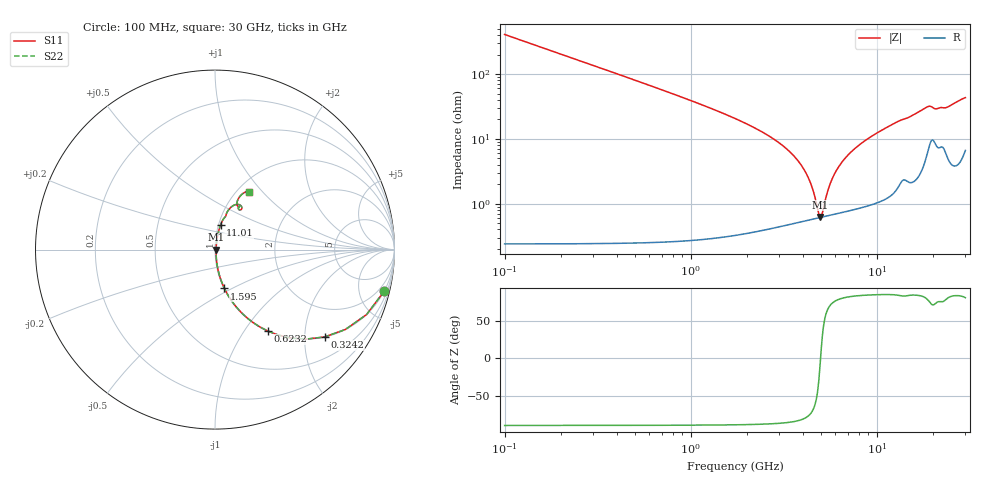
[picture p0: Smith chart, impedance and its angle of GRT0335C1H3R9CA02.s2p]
!Murata Part Number: GRT0335C1H3R9CA02
!These Parameters are Measured in Series Mode Connection
!Data Generated on Jun 19, 2026
!  o--ll--o
!Port1  Port2
!  o------o
!Operation Temp=25[degC], DC Bias Voltage=0[V]
!Freq. Start=100[MHz] Stop=30[GHz] 401[Steps]
# Hz S RI R 50
!Freq.(Hz) S11(Real) S11(Imag) S21(Real) S21(Imag) S12(Real) S12(Imag) S22(Real) S22(Imag)
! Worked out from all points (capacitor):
!   401 points, 100 MHz to 30 GHz, reference 50 ohm
!   read as one part in series: C = 3.9 pF near 249.5 MHz
!   lowest |Z| = 621 mohm at 4.959 GHz (marker M1)
!   series resonance near 4.994 GHz, so ESL is about 260 pH
!   S11 on the Smith chart (normalised r, x): 100 MHz: 1.00, -8.16; 324.2 MHz: 1.00, -2.51; 623.2 MHz: 1.01, -1.29; 1.595 GHz: 1.01, -0.46; 11.01 GHz: 1.02, +0.29; 30 GHz: 1.13, +0.85
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1e8  0.9432 -0.2312  0.0568 0.2312  0.0568 0.2312  0.9432 -0.2312
3.2425e8  0.6107 -0.4866  0.3893 0.4866  0.3893 0.4866  0.6107 -0.4866
6.2325e8  0.294 -0.4536  0.706 0.4536  0.706 0.4536  0.294 -0.4536
9.97e8  0.1351 -0.3385  0.8649 0.3385  0.8649 0.3385  0.1351 -0.3385
1.595e9  0.0525 -0.2162  0.9475 0.2162  0.9475 0.2162  0.0525 -0.2162
3.16475e9  0.0103 -0.0753  0.9897 0.0753  0.9897 0.0753  0.0103 -0.0753
3.91225e9  0.00676 -0.0393  0.9932 0.0393  0.9932 0.0393  0.00676 -0.0393
4.36075e9  0.00606 -0.0217  0.9939 0.0217  0.9939 0.0217  0.00606 -0.0217
4.80925e9  0.00599 -0.00601  0.994 0.00601  0.994 0.00601  0.00599 -0.00601
4.95875e9  0.00607 -0.00114  0.9939 0.00114  0.9939 0.00114  0.00607 -0.00114
5.10825e9  0.0062 0.00359  0.9938 -0.00359  0.9938 -0.00359  0.0062 0.00359
5.482e9  0.0067 0.0148  0.9933 -0.0148  0.9933 -0.0148  0.0067 0.0148
5.70625e9  0.0071 0.0212  0.9929 -0.0212  0.9929 -0.0212  0.0071 0.0212
6.60325e9  0.00934 0.0448  0.9907 -0.0448  0.9907 -0.0448  0.00934 0.0448
8.0235e9  0.0145 0.0775  0.9855 -0.0775  0.9855 -0.0775  0.0145 0.0775
1.01165e10  0.025 0.12  0.975 -0.12  0.975 -0.12  0.025 0.12
1.10135e10  0.0308 0.1371  0.9692 -0.1371  0.9692 -0.1371  0.0308 0.1371
1.505e10  0.0633 0.1996  0.9367 -0.1996  0.9367 -0.1996  0.0633 0.1996
1.856325e10  0.124 0.2519  0.876 -0.2519  0.876 -0.2519  0.124 0.2519
2.005825e10  0.1461 0.2237  0.8539 -0.2237  0.8539 -0.2237  0.1461 0.2237
2.50665e10  0.1261 0.275  0.8739 -0.275  0.8739 -0.275  0.1261 0.275
3e10  0.1919 0.3237  0.8081 -0.3237  0.8081 -0.3237  0.1919 0.3237
